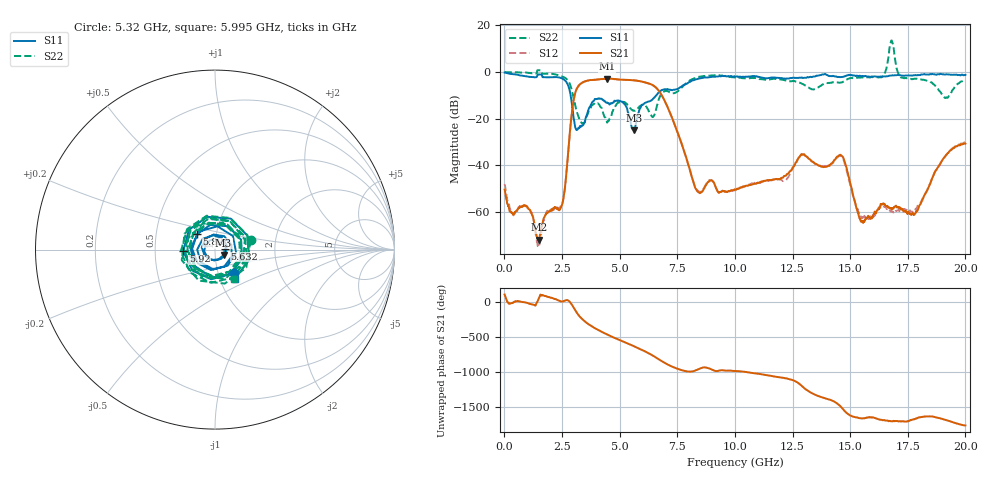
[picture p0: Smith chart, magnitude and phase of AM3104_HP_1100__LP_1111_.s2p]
!Created with skrf (http://scikit-rf.org).
# Hz S RI R 50.0
!freq ReS11 ImS11 ReS21 ImS21 ReS12 ImS12 ReS22 ImS22
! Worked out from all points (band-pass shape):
!   1601 points, 10 MHz to 20 GHz, reference 50 ohm
!   highest |S21| = -2.87 dB at 4.458 GHz (marker M1); lowest = -72.0 dB at 1.497 GHz (marker M2)
!   |S21| within 3 dB of the highest: 3.224 GHz to 6.472 GHz (3.248 GHz wide, 67 % of centre)
!   lowest |S11| = -25.0 dB at 5.645 GHz (marker M3), VSWR 1.12, Z = 54.9 - j3.28 ohm
!   |S11| at or under -10 dB: 2.874 GHz to 6.596 GHz (3.722 GHz wide, 78.6 % of centre)
!   |S22| runs from -22.2 to 13.5 dB; largest |S21 - S12| = 0.083
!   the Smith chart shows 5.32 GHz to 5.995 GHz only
!   S11 on the Smith chart (normalised r, x): 5.32 GHz: 1.19, -0.32; 5.632 GHz: 1.12, +0.01; 5.82 GHz: 0.81, +0.14; 5.92 GHz: 0.70, -0.01; 5.995 GHz: 1.17, -0.40
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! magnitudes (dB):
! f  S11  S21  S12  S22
! 10 MHz  -0.2  -50.5  -48.1  -0.1
! 1.497 GHz  -1.0  -72.0  -74.3  0.8
! 2.496 GHz  -2.7  -57.1  -57.1  -1.9
! 2.996 GHz  -19.1  -12.5  -12.5  -10.9
! 3.346 GHz  -23.2  -4.8  -4.8  -21.8
! 4.458 GHz  -13.1  -2.9  -2.9  -21.7
! 5.32 GHz  -15.5  -3.4  -3.4  -13.7
! 5.632 GHz  -25.0  -3.6  -3.6  -16.6
! 5.645 GHz  -25.0  -3.6  -3.6  -16.7
! 5.82 GHz  -17.6  -3.8  -3.9  -15.3
! 5.92 GHz  -15.0  -4.0  -4.0  -14.4
! 5.995 GHz  -14.1  -4.2  -4.2  -14.1
! 6.682 GHz  -8.9  -7.8  -7.8  -12.3
! 8.368 GHz  -3.0  -51.3  -50.8  -2.2
! 10.01 GHz  -2.0  -50.6  -50.8  -2.4
! 13.34 GHz  -2.2  -38.4  -38.4  -7.4
! 14.65 GHz  -2.2  -36.2  -36.6  -4.4
! 15.5 GHz  -1.8  -64.3  -62.8  -2.3
! 16.68 GHz  -1.7  -58.1  -59.5  7.2
! 17.83 GHz  -1.3  -60.7  -58.9  -2.9
! 19.16 GHz  -1.0  -35.6  -35.7  -10.9
! 20 GHz  -1.3  -30.8  -30.0  -3.3
